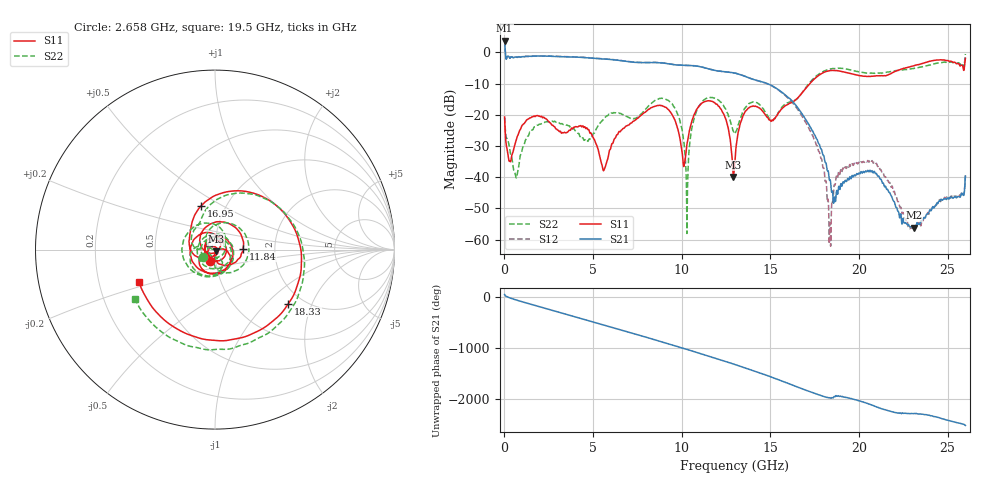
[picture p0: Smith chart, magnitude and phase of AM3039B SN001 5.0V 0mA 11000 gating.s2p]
!Agilent Technologies,E8364B,MY43040894,A.07.50.67
!Agilent E8364B: A.07.50.67
!Date: Tuesday, June 28, 2016 08:09:55
!Correction: S11(Full 2 Port(1,2))
!S21(Full 2 Port(1,2))
!S12(Full 2 Port(1,2))
!S22(Full 2 Port(1,2))
!S2P File: Measurements: S11, S21, S12, S22:
# Hz S  dB  R 50
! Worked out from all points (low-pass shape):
!   1601 points, 10 MHz to 26 GHz, reference 50 ohm
!   highest |S21| = 3.75 dB at 10 MHz (marker M1); lowest = -56.1 dB at 23.09 GHz (marker M2)
!   |S21| within 3 dB of the highest: start of sweep to 43.94 MHz
!   lowest |S11| = -39.9 dB at 12.91 GHz (marker M3), VSWR 1.02, Z = 50.5 - j0.887 ohm
!   |S11| at or under -10 dB: start of sweep to 17.23 GHz
!   |S22| runs from -58.0 to -0.5 dB; largest |S21 - S12| = 0.025
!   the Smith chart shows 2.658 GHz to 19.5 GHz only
!   S11 on the Smith chart (normalised r, x): 2.658 GHz: 0.93, -0.12; 11.84 GHz: 1.37, +0.02; 16.95 GHz: 0.77, +0.40; 18.33 GHz: 1.69, -1.37; 19.5 GHz: 0.38, -0.18
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1e7  -20.71 63.1  3.75 40.9  3.82 41.7  -20.93 17.8
9.358938e8  -24.21 94.1  -1.49 -93.8  -1.45 -93.7  -32.56 100.6
1.796812e9  -20.27 1.8  -1.17 179.4  -1.13 179.6  -23.46 -21.9
2.657731e9  -23.17 -115.6  -1.26 94.2  -1.19 94.4  -22.09 -148.2
3.534894e9  -25.65 79.3  -1.45 8.4  -1.38 8.6  -23.29 72.0
4.347081e9  -23.77 -57.5  -1.59 -72.3  -1.54 -72.2  -26.96 -74.2
5.33795e9  -32.37 138.8  -2.02 -171.1  -1.96 -171.0  -23.35 52.7
6.263844e9  -27.35 -124.1  -2.42 95.4  -2.37 95.9  -19.37 -97.6
7.303444e9  -21.98 62.7  -3.17 -8.0  -3.12 -7.6  -21.17 78.1
8.684162e9  -17.03 -142.6  -3.29 -147.5  -3.23 -146.9  -14.96 -156.0
1.029229e10  -29.49 -141.7  -4.18 45.4  -4.16 45.9  -58.01 -86.6
1.183545e10  -16.05 2.1  -5.73 -122.4  -5.72 -121.8  -14.62 -12.6
1.290754e10  -39.90 -60.3  -6.53 119.6  -6.51 120.3  -25.21 -87.8
1.3005e10  -34.78 2.3  -6.64 108.3  -6.65 109.0  -26.00 -74.1
1.695223e10  -11.84 107.4  -21.18 -28.7  -22.09 -27.7  -11.64 92.7
1.734208e10  -9.29 72.2  -24.89 -77.0  -26.33 -76.3  -8.88 60.3
1.833295e10  -5.89 -36.4  -40.94 176.4  -60.62 -118.2  -5.39 -37.2
1.95025e10  -6.74 -156.6  -39.90 162.1  -36.04 -179.4  -5.60 -148.3
2.167916e10  -7.10 37.8  -44.78 -79.5  -41.67 -83.2  -6.25 46.4
2.309237e10  -4.30 -69.5  -56.14 -133.2  -55.55 -146.7  -5.14 -59.2
2.453806e10  -2.38 172.7  -47.67 141.7  -47.17 139.2  -3.31 -169.7
2.6e10  -1.91 1.9  -39.71 -6.5  -39.30 -5.5  -0.51 35.5
